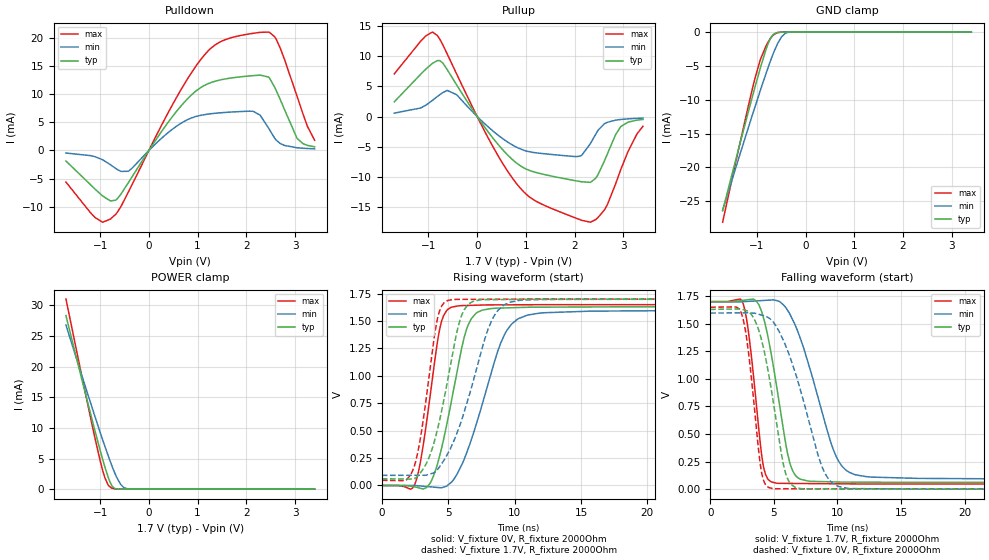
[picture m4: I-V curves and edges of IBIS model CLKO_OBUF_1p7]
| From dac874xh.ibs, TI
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|   CLKO_OBUF_1p7 Model
[Model]   CLKO_OBUF_1p7
Model_type   3-state
Polarity   Non-Inverting
Vmeas = 0.85
Vref = 0
Cref = 2pF
Rref = 100000
|   typ   min   max
C_comp   9.28911E-13   6.32633E-13   9.81634E-13
| Where nom  PVT is Nominal Process, 1.7V, 27C
|   Fast PVT is Strong Process,  1.701V, -40C
|   Slow PVT is Weak Process,   1.699V, 150C
[Voltage Range]   1.7   1.699   1.701
[Temperature Range]   27   150   -40
[Pullup Reference]   1.7   1.699   1.701
[Pulldown Reference]   0   0   -0
[Power Clamp Reference]   1.7   1.699   1.701
[GND Clamp Reference]   0   0   0
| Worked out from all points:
|   slope of the pulldown table from 0 to 0.255 V, typ, clamps not added: 76.9 ohm
|   slope of the pullup table from 0 to 0.255 V, typ, clamps not added: 88.8 ohm
|   GND clamp passes 1 mA (typ) near -0.72 V on its own axis
|   POWER clamp passes 1 mA (typ) near -0.79 V on its own axis
|   falling waveform, V_fixture 1.7V, R_fixture 2000Ohm: 20-80 % time 1.42ns typ, 2.46ns min, 903ps max; typ from 1.7 V to 0.061 V
|   rising waveform, V_fixture 0V, R_fixture 2000Ohm: 20-80 % time 1.64ns typ, 2.43ns min, 1.13ns max; typ from 0 V to 1.63 V
|   rising waveform, V_fixture 1.7V, R_fixture 2000Ohm: 20-80 % time 1.68ns typ, 2.42ns min, 1.14ns max; typ from 0.061 V to 1.7 V
|   falling waveform, V_fixture 0V, R_fixture 2000Ohm: 20-80 % time 1.45ns typ, 2.44ns min, 907ps max; typ from 1.63 V to 0 V
[Pulldown]
|   Voltage   I(typ)   I(min)   I(max)
-1.7V     -1.875mA   -453.2uA   -5.626mA
-1.098V   -6.932mA   -1.123mA   -11.97mA
-787.1mV  -8.98mA    -2.542mA   -12.21mA
-419.9mV  -5.729mA   -3.705mA   -7.404mA
472.6mV   5.918mA    3.723mA    7.969mA
1.059V    11.19mA    6.261mA    16.15mA
1.442V    12.53mA    6.699mA    19.25mA
2.054V    13.27mA    6.999mA    20.76mA
2.457V    13.09mA    3.968mA    21.1mA
2.604V    10.83mA    1.929mA    19.93mA
3.043V    2.123mA    485.6uA    9.572mA
3.4V      657.2uA    296.4uA    1.815mA
[GND Clamp]
|   Voltage   I(typ)   I(min)   I(max)
-1.7V     -26.42mA   -26.34mA   -28.11mA
-1.175V   -11.84mA   -14.18mA   -10.98mA
-1.032V   -8.019mA   -10.96mA   -6.715mA
-924.8mV  -5.268mA   -8.587mA   -4.057mA
-812.6mV  -2.631mA   -6.178mA   -2.096mA
-720.8mV  -959.4uA   -4.305mA   -938.1uA
-649.4mV  -283.4uA   -2.961mA   -382.8uA
-567.8mV  -51.5uA    -1.638mA   -81.02uA
-491.3mV  -8.113uA   -704.9uA   -11.75uA
-419.9mV  -1.091uA   -201.5uA   -1.26uA
-338.3mV  -67.86nA   -27.66uA   -43.06nA
3.4V      0A         0A         0A
[Pullup]
|   Voltage   I(typ)   I(min)   I(max)
-1.7V     2.441mA    567.1uA    7.066mA
-1.052V   7.868mA    1.882mA    13.39mA
-817.7mV  9.268mA    3.311mA    13.45mA
-419.9mV  5.227mA    3.61mA     7.031mA
324.7mV   -3.6mA     -2.412mA   -5.03mA
819.4mV   -7.789mA   -5.134mA   -11.25mA
1.192V    -9.249mA   -6.007mA   -13.98mA
2.054V    -10.7mA    -6.642mA   -16.94mA
2.324V    -10.91mA   -4.471mA   -17.53mA
2.61V     -7.36mA    -1.199mA   -15.49mA
2.946V    -1.654mA   -486.9uA   -8.752mA
3.4V      -488.8uA   -267.3uA   -1.623mA
[POWER Clamp]
|   Voltage   I(typ)   I(min)   I(max)
-1.7V     28.29mA    26.76mA    31mA
-1.353V   17.22mA    17.99mA    17.59mA
-1.144V   10.7mA     12.8mA     9.741mA
-1.001V   6.412mA    9.337mA    4.732mA
-899.3mV  3.552mA    6.937mA    1.813mA
-838.1mV  2.025mA    5.544mA    739.3uA
-771.8mV  741.3uA    4.1mA      210.3uA
-705.5mV  136.6uA    2.761mA    50.43uA
-583.1mV  3.076uA    836.9uA    1.89uA
-511.7mV  348.6nA    247.9uA    166.1nA
-419.9mV  10.3nA     26.98uA    0A
3.4V      0A         0A         0A
[Ramp]
R_load = 2000
|   typ   min   max
dV/dt_r   0.97813/1.63672e-09   0.958223/2.42744e-09   0.990052/1.13192e-09
dV/dt_f   0.98325/1.41697e-09   0.964063/2.46106e-09   0.99248/9.03504e-10
[Falling Waveform]
V_fixture = 1.7V
V_fixture_min = 1.699V
V_fixture_max = 1.701V
R_fixture = 2000Ohm
C_fixture = 0F
|   Time   V(typ)   V(min)   V(max)
0s        1.7V       1.699V     1.701V
2.577ns   1.712V     1.7V       1.686V
3.089ns   1.72V      1.704V     1.353V
4.159ns   1.565V     1.711V     223.4mV
4.804ns   1.221V     1.716V     65.32mV
6.077ns   326.1mV    1.623V     52.32mV
6.645ns   133.7mV    1.498V     51.79mV
9.658ns   66.02mV    364.7mV    48.98mV
10.96ns   63.81mV    151.4mV    47.78mV
30ns      61.25mV    92.23mV    46.87mV
[Rising Waveform]
V_fixture = 0V
V_fixture_min = 0V
V_fixture_max = 0V
R_fixture = 2000Ohm
C_fixture = 0F
|   Time   V(typ)   V(min)   V(max)
0s        882.7pV    20.74nV    380.6pV
2.498ns   -13.05mV   -591.1uV   15.47mV
3.612ns   16.49mV    -12.23mV   795.7mV
4.41ns    297.4mV    -20.61mV   1.457V
5.226ns   761.7mV    28.18mV    1.626V
6.201ns   1.351V     239.2mV    1.642V
6.744ns   1.523V     419.4mV    1.644V
8.94ns    1.619V     1.296V     1.648V
10.3ns    1.624V     1.523V     1.649V
30ns      1.63V      1.597V     1.65V
[Rising Waveform]
V_fixture = 1.7V
V_fixture_min = 1.699V
V_fixture_max = 1.701V
R_fixture = 2000Ohm
C_fixture = 0F
|   Time   V(typ)   V(min)   V(max)
0s        61.25mV    92.23mV    46.87mV
1.759ns   58.63mV    92.58mV    43.84mV
2.384ns   61.75mV    92.7mV     154.4mV
2.998ns   131mV      92.83mV    502.8mV
4.196ns   515.2mV    146.7mV    1.527V
4.96ns    962.9mV    289.3mV    1.688V
6.201ns   1.603V     671.3mV    1.698V
8.002ns   1.696V     1.426V     1.699V
9.224ns   1.697V     1.648V     1.7V
30ns      1.7V       1.699V     1.701V
[Falling Waveform]
|Gnd
V_fixture = 0V
V_fixture_min = 0V
V_fixture_max = 0V
R_fixture = 2000Ohm
C_fixture = 0F
|   Time   V(typ)   V(min)   V(max)
0s        1.63V      1.597V     1.65V
2.498ns   1.63V      1.599V     1.58V
2.998ns   1.61V      1.6V       1.251V
3.944ns   1.392V     1.582V     219.2mV
4.579ns   1.054V     1.554V     15.68mV
5.631ns   298.9mV    1.379V     3.385mV
6.201ns   67.89mV    1.222V     3.369mV
8.653ns   2.771mV    246.1mV    3.299mV
9.788ns   1.973mV    41.1mV     3.267mV
30ns      -115.1pV   20.75nV    380.2pV
